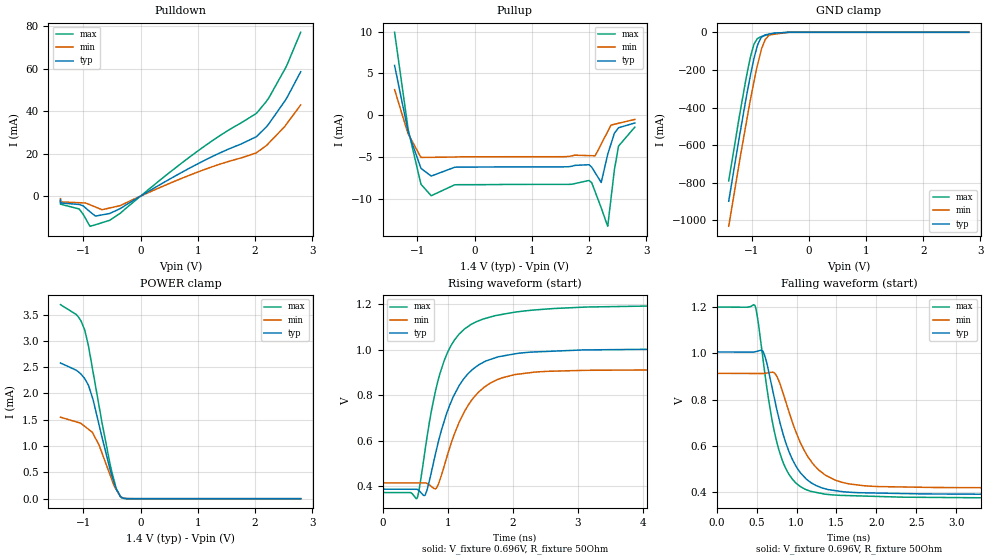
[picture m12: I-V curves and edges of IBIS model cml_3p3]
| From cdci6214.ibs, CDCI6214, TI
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|   cml_3p3 Model
[Model]   cml_3p3
Model_type   3-state
Polarity   Non-Inverting
Vmeas = 0.7
Vref = 0.696
Cref = 2pF
Rref = 50
|   typ   min   max
C_comp   6.977E-12   6.849E-12   7.106E-12
|  Where Nom  PVT is Nominal Process, 1.4V,   32C
|   Fast PVT is Strong Process,  1.43V,  -35C
|   Slow PVT is Weak Process,   1.39V,  110C
[Voltage Range]   1.4   1.39   1.43
|Junction Temperature
[Temperature Range]   32   110   -35
[Pullup Reference]   1.4   1.39   1.43
[Pulldown Reference]   0   0   0
[Power Clamp Reference]   1.4   1.39   1.43
[GND Clamp Reference]   0   0   0
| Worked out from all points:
|   slope of the pulldown table from 0 to 0.21 V, typ, clamps not added: 62.5 ohm
|   POWER clamp passes 1 mA (typ) near -0.64 V on its own axis
|   falling waveform, V_fixture 0.696V, R_fixture 50Ohm: 20-80 % time 321ps typ, 382ps min, 265ps max; typ from 1 V to 0.388 V
|   rising waveform, V_fixture 0.696V, R_fixture 50Ohm: 20-80 % time 485ps typ, 499ps min, 441ps max; typ from 0.388 V to 1 V
[Pulldown]
|   Voltage   I(typ)   I(min)   I(max)
-1.4V     -1.635mA   -1.155mA   -2.213mA
-1.399V   -3.204mA   -2.715mA   -3.792mA
-1.072V   -3.917mA   -3.1mA     -6.039mA
-884.5mV  -7.34mA    -4.056mA   -14.2mA
-789.2mV  -9.391mA   -5.11mA    -13.47mA
-673.3mV  -8.826mA   -6.392mA   -12.5mA
-349.9mV  -5.8mA     -4.435mA   -7.968mA
966.8mV   14.73mA    11mA       20.57mA
2.033V    28.16mA    20.56mA    39.16mA
2.248V    34.2mA     25.11mA    46.47mA
2.536V    45.3mA     33.33mA    60.39mA
2.8V      58.53mA    42.95mA    77.13mA
[GND Clamp]
|   Voltage   I(typ)   I(min)   I(max)
-1.4V     -898.3mA   -1.032A    -790.1mA
-1.226V   -578.5mA   -714.2mA   -469.3mA
-1.103V   -362.2mA   -497.9mA   -255.7mA
-1.017V   -224mA     -353.6mA   -127.9mA
-965.2mV  -148.6mA   -273.5mA   -70.11mA
-914.4mV  -88.51mA   -195.4mA   -41.08mA
-889.6mV  -63.24mA   -165.3mA   -31.84mA
-824.5mV  -25.66mA   -86.62mA   -22.31mA
-760.2mV  -13.72mA   -37.99mA   -16.45mA
-688mV    -9.205mA   -13.77mA   -11.1mA
-349.5mV  -107.1uA   -120.1uA   -86.75uA
2.8V      0A         0A         0A
[Pullup]
|   Voltage   I(typ)   I(min)   I(max)
-1.4V     5.953mA    3.06mA     9.924mA
-1.161V   -2.044mA   -2.257mA   -1.769mA
-941.2mV  -6.326mA   -5.047mA   -8.207mA
-759.8mV  -7.297mA   -5.053mA   -9.653mA
-349.9mV  -6.244mA   -5.02mA    -8.346mA
2.001V    -5.939mA   -4.847mA   -7.819mA
2.107V    -6.898mA   -4.867mA   -9.181mA
2.213V    -8.064mA   -3.464mA   -11.1mA
2.326V    -4.697mA   -1.961mA   -13.31mA
2.443V    -2.172mA   -1.092mA   -6.561mA
2.516V    -1.51mA    -973.7uA   -3.706mA
2.8V      -938.8uA   -511.8uA   -1.44mA
[POWER Clamp]
|   Voltage   I(typ)   I(min)   I(max)
-1.4V     2.58mA     1.55mA     3.689mA
-1.124V   2.443mA    1.46mA     3.503mA
-1.04V    2.367mA    1.431mA    3.377mA
-977.3mV  2.286mA    1.377mA    3.212mA
-915.6mV  2.166mA    1.324mA    2.931mA
-827.4mV  1.873mA    1.231mA    2.392mA
-726.2mV  1.408mA    1.022mA    1.769mA
-533mV    556.4uA    452.5uA    659.8uA
-432.2mV  204.7uA    186.2uA    221.7uA
-340.2mV  32.23uA    34.76uA    25.32uA
-191.1mV  312.7nA    713.9nA    63.12nA
2.8V      0A         0A         0A
[Ramp]
R_load = 50
|   typ   min   max
dV/dt_r   0.370478/4.85519e-10   0.29842/4.99664e-10   0.495516/4.41185e-10
dV/dt_f   0.370475/3.20544e-10   0.29842/3.81393e-10   0.495515/2.64267e-10
[Falling Waveform]
V_fixture = 0.696V
V_fixture_min = 0.664V
V_fixture_max = 0.785V
R_fixture = 50Ohm
C_fixture = 0F
|   Time   V(typ)   V(min)   V(max)
0s        1.005V     913.1mV    1.199V
478.7ps   1.006V     912.7mV    1.206V
601.3ps   989.6mV    913.4mV    918.6mV
704.1ps   835.8mV    917.6mV    692.8mV
816.4ps   670.5mV    843.7mV    543.7mV
1.028ns   494.6mV    631.1mV    430.8mV
1.361ns   415.5mV    474.6mV    392.3mV
1.84ns    398.5mV    429mV      384.5mV
2.737ns   393.4mV    421.3mV    378.5mV
20ns      387.9mV    415.7mV    373.1mV
[Rising Waveform]
V_fixture = 0.696V
V_fixture_min = 0.664V
V_fixture_max = 0.785V
R_fixture = 50Ohm
C_fixture = 0F
|   Time   V(typ)   V(min)   V(max)
0s        387.9mV    415.7mV    373.1mV
535.1ps   386.4mV    415.4mV    351.1mV
657.2ps   363.6mV    415.4mV    566.7mV
825.9ps   558.2mV    391.9mV    834.4mV
946.7ps   686.1mV    489mV      952.7mV
1.106ns   804.5mV    631.6mV    1.044V
1.479ns   934.5mV    815.5mV    1.128V
2.031ns   982.7mV    891.5mV    1.166V
4.931ns   1.005V     912.9mV    1.197V
20ns      1.005V     913.1mV    1.199V
